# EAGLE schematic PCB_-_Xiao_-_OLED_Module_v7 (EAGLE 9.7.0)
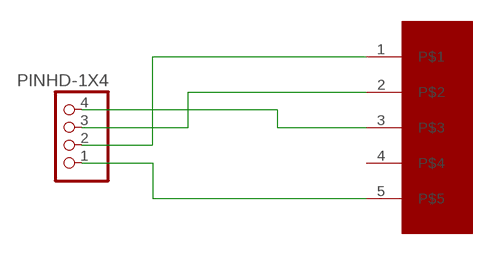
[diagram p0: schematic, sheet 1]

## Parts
JP1  PINHD-1X4  [1X04]
U$1  1X5_PAD_SMD  [1X05SMD]

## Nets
N$1: JP1.1 U$1.5
N$2: JP1.2 U$1.1
N$3: JP1.3 U$1.2
N$4: JP1.4 U$1.3
Unconnected: U$1.4

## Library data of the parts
JP1 = Connector:PINHD-1X4: PIN HEADER; CATEGORY: Headers; DESCRIPTION: Header-Straight-4 Position; PACKAGE_TYPE: THT; PITCH: 0.100" (2.54mm); SUBCATEGORY: Headers-Male Pins; TYPE: Board to Board or Cable-Unshrouded-Through Hole-Straight
U$1 = Carl_Lib:1X5_PAD_SMD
